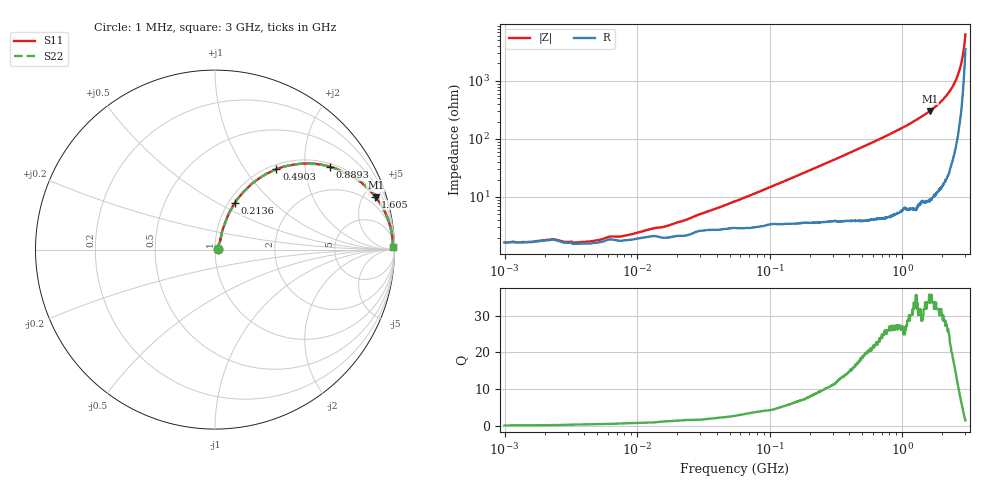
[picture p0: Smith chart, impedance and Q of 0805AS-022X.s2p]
!s-Parameter Generated by FASTRON Sdn. Bhd.
!FASTRON P/N : 0805AS-022X
!Keysight Technologies: E4991B_MY54100416_A.01.15
!Date: Mon Jun 15 12:49:37 2026
!Version  :Rev01  Mon Jun 15 12:49:37 2026
!Data & Calibration Information:
!Freq  S11  S21  S12  S22
!PortZ  Port1:50+j0  Port2:50+j0
!When reading reference impedance value at option line is always used.
! Remarks : This data is being provided solely for informational purposes.
# Hz S dB R 50
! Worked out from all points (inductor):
!   1601 points, 1 MHz to 3 GHz, reference 50 ohm
!   read as one part in series: L = 22.8 nH near 60.54 MHz
!   highest Q = 33.7 at 1.621 GHz (marker M1), where L = 29.9 nH
!   S11 on the Smith chart (normalised r, x): 1 MHz: 1.03, +0.00; 213.6 MHz: 1.07, +0.61; 490.3 MHz: 1.08, +1.41; 889.3 MHz: 1.10, +2.70; 1.605 GHz: 1.18, +5.98; 3 GHz: open
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1000000  -35.80 5.1  -0.14 -0.1  -0.14 -0.1  -35.80 5.1
2306346  -34.70 10.4  -0.16 -0.2  -0.16 -0.2  -34.70 10.4
2845765  -35.60 14.4  -0.14 -0.2  -0.14 -0.2  -35.60 14.4
3804036  -35.70 19.5  -0.14 -0.3  -0.14 -0.3  -35.70 19.5
7819618  -33.60 32.5  -0.15 -0.7  -0.15 -0.7  -33.60 32.5
1.447069e7  -30.70 44.7  -0.18 -1.2  -0.18 -1.2  -30.70 44.7
2.304607e7  -28.20 55.4  -0.19 -1.9  -0.19 -1.9  -28.20 55.4
5.504702e7  -21.70 65.3  -0.28 -4.4  -0.28 -4.4  -21.70 65.3
1.098084e8  -16.30 69.1  -0.39 -8.6  -0.39 -8.6  -16.30 69.1
2.083556e8  -11.10 67.1  -0.65 -16.0  -0.65 -16.0  -11.10 67.1
2.136344e8  -10.90 66.9  -0.67 -16.4  -0.67 -16.4  -10.90 66.9
3.351655e8  -7.54 60.7  -1.16 -24.8  -1.16 -24.8  -7.54 60.7
4.902556e8  -4.98 52.6  -1.98 -34.2  -1.98 -34.2  -4.98 52.6
7.925923e8  -2.49 39.2  -3.98 -48.6  -3.98 -48.6  -2.49 39.2
8.892696e8  -2.05 35.7  -4.67 -52.2  -4.67 -52.2  -2.05 35.7
1.206698e9  -1.11 26.6  -6.97 -61.6  -6.97 -61.6  -1.11 26.6
1.604986e9  -0.54 18.3  -10.10 -70.0  -10.10 -70.0  -0.54 18.3
1.621129e9  -0.52 18.0  -10.20 -70.3  -10.20 -70.3  -0.52 18.0
2.071593e9  -0.23 11.2  -14.20 -76.8  -14.20 -76.8  -0.23 11.2
2.480502e9  -0.11 6.2  -19.40 -80.3  -19.40 -80.3  -0.11 6.2
2.741597e9  -0.08 3.3  -24.60 -79.4  -24.60 -79.4  -0.08 3.3
3e9  -0.08 0.7  -36.10 -55.2  -36.10 -55.2  -0.08 0.7
